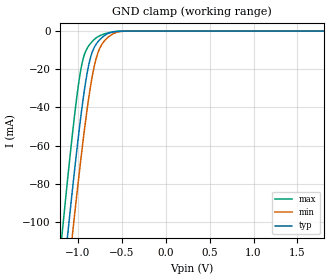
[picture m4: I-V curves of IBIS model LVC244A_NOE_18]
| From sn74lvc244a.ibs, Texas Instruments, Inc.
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[Model]   LVC244A_NOE_18
Model_type  Input
Vinl=0.5775
Vinh=1.2675
| variable   typ   min   max
C_comp   2.67pF   2.18pF   3.26pF
[Temperature Range]   40   100   -40
| Ambient temperature   25   85   -40
[Voltage range]   1.8   1.65   1.95
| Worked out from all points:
|   GND clamp passes 1 mA (typ) near -0.64 V on its own axis
[GND Clamp]
| LVC244A_NOE_18
|   Voltage   I(typ)   I(min)   I(max)
-5.5V     -2.303A    -2.296A    -2.31A
-1.18V    -134.8mA   -158.2mA   -105.7mA
-1.115V   -105.6mA   -129.2mA   -76.15mA
-1.07V    -85.97mA   -109.6mA   -56.7mA
-1.055V   -79.59mA   -103.1mA   -50.5mA
-965mV    -43.83mA   -66.22mA   -19.51mA
-875mV    -17.2mA    -34.23mA   -7.542mA
-820mV    -9.056mA   -19.54mA   -4.611mA
-775mV    -5.72mA    -11.65mA   -3.005mA
-645mV    -1.023mA   -2.792mA   -765uA
-435mV    -12.49uA   -27.87uA   -3.401uA
1.8V      41.95pA    147.7pA    23.47pA
